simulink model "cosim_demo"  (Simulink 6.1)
settings: Solver=ode45  StartTime=0.0  StopTime=300  RelTol=1e-3
undefined symbols (not defined in the file or in its folder): cosim_demo_src_clk_wrapper, Double, n, netlist, simulink
libraries: xbsIndex_r3 x9

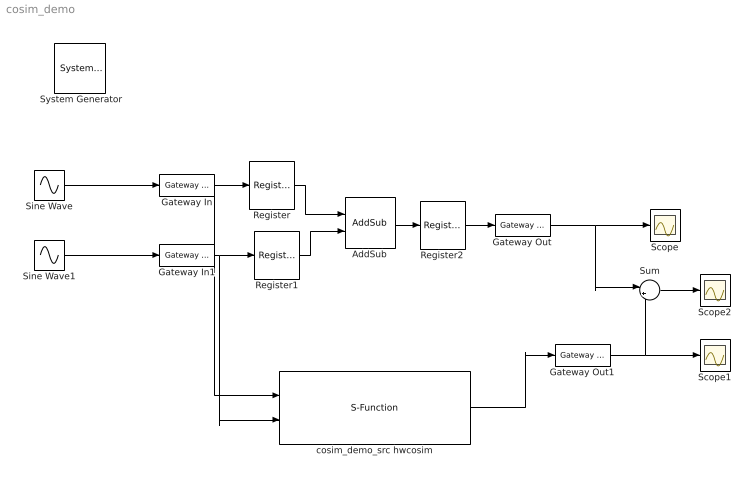
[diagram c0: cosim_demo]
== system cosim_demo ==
  " System Generator" : xbsIndex_r3/ System Generator  Tag=genX  xilinxfamily=Virtex2P  part=xc2vp7  speed=-6  package=ff896  synthesis_tool=Synplify Pro  directory=./netlist  testbench=off  simulink_period=1  sysclk_period=25  incr_netlist=off  trim_vbits=Everywhere in SubSystem  dbl_ovrd=According to Block Masks  core_generation=According to Block Masks  run_coregen=off  deprecated_control=off  eval_field=0
  AddSub : xbsIndex_r3/AddSub  mode=Addition  precision=Full  arith_type=Unsigned  n_bits=8  bin_pt=2  quantization=Truncate  overflow=Wrap  latency=0  explicit_period=off  period=1  use_carryin=off  use_carryout=off  en=off  dbl_ovrd=off  show_param=off  use_core=on  pipeline=off  use_rpm=off  gen_core=off
  Gateway In : xbsIndex_r3/Gateway In  arith_type="Signed  (2's comp)"  n_bits=12  bin_pt=0  quantization=Truncate  overflow=Wrap  period=1  timing_constraint=None  locs_specified=off  LOCs={}  needs_fixed_name=off  dbl_ovrd=off  show_param=off
  Gateway In1 : xbsIndex_r3/Gateway In  arith_type="Signed  (2's comp)"  n_bits=12  bin_pt=0  quantization=Truncate  overflow=Wrap  period=1  timing_constraint=None  locs_specified=off  LOCs={}  needs_fixed_name=off  dbl_ovrd=off  show_param=off
  Gateway Out : xbsIndex_r3/Gateway Out  output_type=Double  nbits=8  bin_pt=6  arith_type=Boolean  quantization=Truncate  overflow=Wrap  hdl_port=on  timing_constraint=None  locs_specified=off  LOCs={}  needs_fixed_name=off  show_param=off
  Gateway Out1 : xbsIndex_r3/Gateway Out  output_type=Double  nbits=8  bin_pt=6  arith_type=Boolean  quantization=Truncate  overflow=Wrap  hdl_port=off  timing_constraint=None  locs_specified=off  LOCs={}  needs_fixed_name=off  show_param=off
  Register : xbsIndex_r3/Register  init=0  reg_only_valid=off  explicit_period=off  period=1  rst=off  en=off  out_en=off  dbl_ovrd=off  show_param=off
  Register1 : xbsIndex_r3/Register  init=0  reg_only_valid=off  explicit_period=off  period=1  rst=off  en=off  out_en=off  dbl_ovrd=off  show_param=off
  Register2 : xbsIndex_r3/Register  init=0  reg_only_valid=off  explicit_period=off  period=1  rst=off  en=off  out_en=off  dbl_ovrd=off  show_param=off
  Scope : Scope
  Scope1 : Scope
  Scope2 : Scope
  Sine Wave : Sin  Amplitude=2000  Frequency=.1  SampleTime=1
  Sine Wave1 : Sin  Amplitude=1000  Frequency=.3  SampleTime=1
  Sum : Sum  Inputs=|+-
  cosim_demo_src hwcosim : S-Function  FunctionName=xlcosim  Parameters=sfcn_mwsv__  mask(Alpha Data ADM-XRC-II Hardware Cosimulation){prtNames={'gateway_in','gateway_in1','gateway_out'}, prtTypes={'Fix_12_0','Fix_12_0','Fix_13_0'}, blkPeriod=1, prtDirs=[0,0,1], prtDataRates=[1,1,1], prtSignalType=Double, bitFileName=n:\simulink\netlist\cosim_demo_src_clk_wrapper.bit, cardIndex=0}
      mask prompts: prtNames "Port Names (specified as cell array of strings)"; prtTypes "Port Types (specified as cell array of strings, eg 'Fix_8_7')"; blkPeriod "Internal Block Period"; prtDirs "Port Directions (specified as vector of integers, eg 'in'= 0 'out'=1)"; prtDataRates "Port Data Rates (specified as vector of integers)"; prtSignalType "Port Signal Type"; bitFileName "Configuration File"; cardIndex "Card Index"
      mask help: Cosimulation for ADM-XRC, ADM-XRC-II, ADM-XPL boards.
      mask init:
      | [bg,fg] = xlcmap('XBlock',1);
      | 
      | iPos = get_param(gcb,'Position');
      | iWidth=iPos(3)-iPos(1); iHeight=iPos(4)-iPos(2);
      | iCx=iWidth/2;
      | iCy=iHeight/2;
      | [logoX, logoY] = xlogo(iPos);
      | 
      | ports = xlPortLabel(prtNames,prtDirs,30);
      | 
      | % assumes the cosim DLL resides in the same
      | % directory as the library containing the
      | % cosim block
      | libDir = which('admxrciip_RunTimeCosim');
      | binDir = fileparts(libDir);
      | %binDir = xlPathToReference;
      | 
      | 
      | % cosim DLL name goes here
      | engineDll = 'XRC_CosimEngine.dll';
      | 
      | % pass all mask workspace variables 
      | % to S-function
      | sfcn_mwsv__ = get_param(gcb, 'MaskWSVariables');
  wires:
  Sine Wave/1 -> Gateway In/1
  Sine Wave1/1 -> Gateway In1/1
  Gateway In/1 -> Register/1, cosim_demo_src hwcosim/1
  Gateway In1/1 -> Register1/1, cosim_demo_src hwcosim/2
  Register/1 -> AddSub/1
  Register1/1 -> AddSub/2
  AddSub/1 -> Register2/1
  Register2/1 -> Gateway Out/1
  Gateway Out/1 -> Scope/1, Sum/1
  Sum/1 -> Scope2/1
  cosim_demo_src hwcosim/1 -> Gateway Out1/1
  Gateway Out1/1 -> Scope1/1, Sum/2
